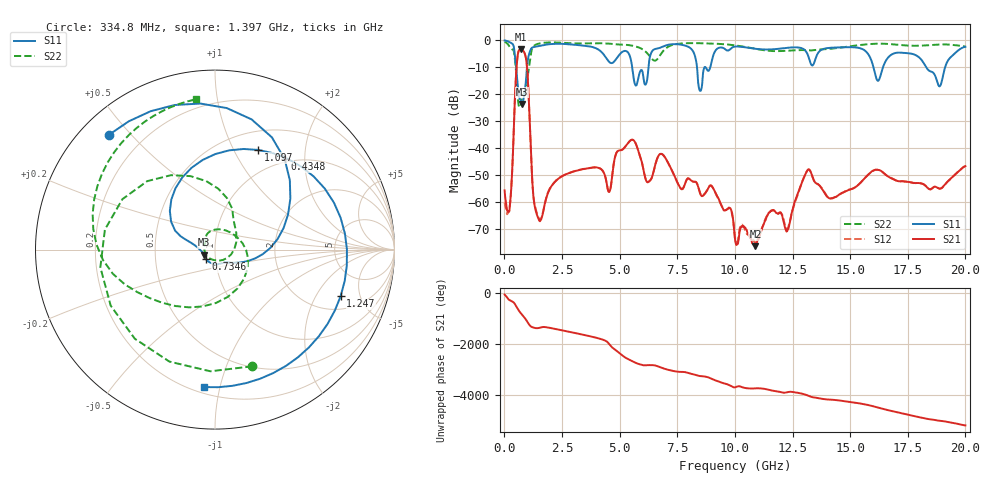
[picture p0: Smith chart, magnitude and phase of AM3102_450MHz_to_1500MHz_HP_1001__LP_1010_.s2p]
!Agilent Technologies,E8364B,MY43040894,A.07.50.67
!Agilent E8364B: A.07.50.67
!Date: Thursday, January 11, 2018 06:04:00
!Correction: S11(Full 2 Port(1,2))
!S21(Full 2 Port(1,2))
!S12(Full 2 Port(1,2))
!S22(Full 2 Port(1,2))
!S2P File: Measurements: S11, S21, S12, S22:
# Hz S  dB  R 50
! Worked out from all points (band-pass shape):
!   1601 points, 10 MHz to 20 GHz, reference 50 ohm
!   highest |S21| = -3.37 dB at 709.6 MHz (marker M1); lowest = -76.3 dB at 10.89 GHz (marker M2)
!   |S21| within 3 dB of the highest: 565.6 MHz to 929.3 MHz (363.7 MHz wide, 48.7 % of centre)
!   lowest |S11| = -23.6 dB at 772.1 MHz (marker M3), VSWR 1.14, Z = 44.3 - j2.52 ohm
!   |S11| at or under -10 dB: 507.4 MHz to 980.2 MHz (472.7 MHz wide, 63.6 % of centre); 5.545 GHz to 6.251 GHz (705.8 MHz wide, 12 % of centre); 18.3 GHz to 19.12 GHz (819.4 MHz wide, 4.38 % of centre)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
!   |S22| runs from -24.8 to -0.5 dB; largest |S21 - S12| = 0.00086
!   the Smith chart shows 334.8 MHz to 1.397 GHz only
!   S11 on the Smith chart (normalised r, x): 334.8 MHz: 0.08, +0.44; 434.8 MHz: 0.95, +1.60; 734.6 MHz: 0.90, -0.10; 1.097 GHz: 0.72, +1.26; 1.247 GHz: 2.81, -3.30; 1.397 GHz: 0.24, -0.90
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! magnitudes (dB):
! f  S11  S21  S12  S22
! 10 MHz  0.0  -55.6  -60.1  -0.5
! 334.8 MHz  -1.2  -49.0  -49.1  -3.3
! 434.8 MHz  -3.9  -26.2  -26.3  -5.4
! 709.6 MHz  -22.2  -3.4  -3.4  -24.3
! 734.6 MHz  -22.8  -3.4  -3.4  -22.8
! 772.1 MHz  -23.6  -3.5  -3.5  -21.1
! 1.097 GHz  -4.4  -29.6  -29.5  -8.3
! 1.247 GHz  -2.5  -56.7  -56.5  -2.4
! 1.397 GHz  -2.3  -64.3  -63.7  -1.5
! 3.346 GHz  -1.9  -47.8  -47.8  -1.2
! 4.545 GHz  -8.0  -56.2  -56.1  -1.2
! 5.707 GHz  -16.8  -38.4  -38.5  -2.3
! 6.219 GHz  -13.0  -52.7  -52.5  -5.0
! 6.682 GHz  -2.9  -42.8  -42.8  -6.4
! 8.081 GHz  -3.0  -51.8  -51.9  -1.0
! 8.493 GHz  -18.8  -56.8  -56.6  -1.1
! 10.01 GHz  -2.3  -73.5  -73.1  -1.9
! 10.89 GHz  -3.1  -76.3  -75.3  -3.2
! 13.34 GHz  -9.3  -49.9  -50.0  -3.7
! 16.68 GHz  -6.1  -50.7  -50.6  -1.4
! 18.88 GHz  -17.1  -55.0  -55.0  -1.6
! 20 GHz  -2.4  -46.7  -46.7  -2.3
